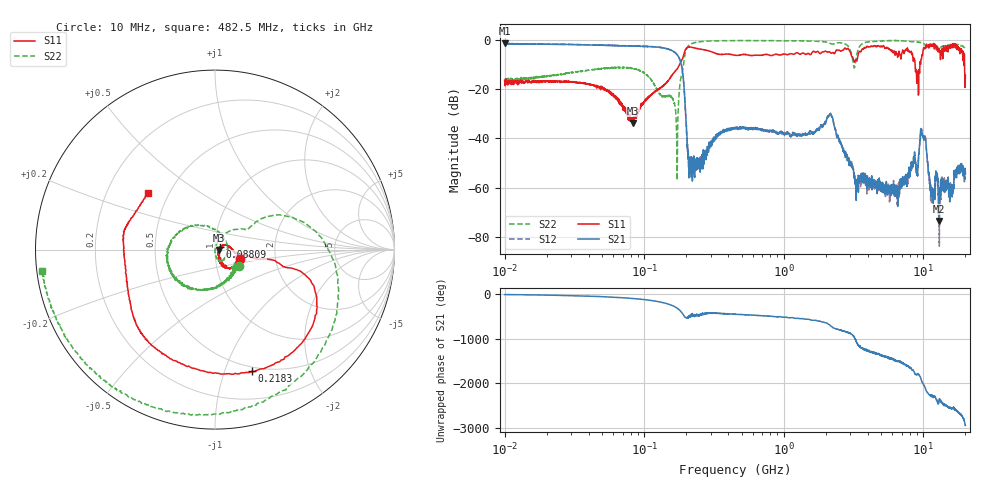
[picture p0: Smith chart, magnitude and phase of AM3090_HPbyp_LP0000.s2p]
# Hz S DB R 50
!freq MagS11 AngS11 MagS21 AngS21 MagS12 AngS12 MagS22 AngS22
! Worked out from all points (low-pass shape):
!   3201 points, 10 MHz to 20 GHz, reference 50 ohm
!   highest |S21| = -1.39 dB at 10.05 MHz (marker M1); lowest = -73.5 dB at 12.95 GHz (marker M2)
!   |S21| within 3 dB of the highest: start of sweep to 158.6 MHz
!   lowest |S11| = -33.7 dB at 82.62 MHz (marker M3), VSWR 1.04, Z = 52.1 - j0.2 ohm
!   |S11| at or under -10 dB: start of sweep to 179.1 MHz; 8.727 GHz to 9.453 GHz (725.5 MHz wide, 7.98 % of centre); 19.73 GHz to end of sweep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
!   |S22| runs from -57.0 to -0.2 dB; largest |S21 - S12| = 0.04
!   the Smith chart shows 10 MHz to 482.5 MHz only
!   S11 on the Smith chart (normalised r, x): 10 MHz: 1.32, -0.13; 88.09 MHz: 1.05, +0.03; 218.3 MHz: 0.46, -1.25; 482.5 MHz: 0.38, +0.32
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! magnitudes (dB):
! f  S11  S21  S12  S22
! 10 MHz  -16.5  -1.5  -1.7  -15.8
! 10.05 MHz  -16.9  -1.4  -1.5  -17.2
! 35.55 MHz  -17.6  -2.0  -1.9  -12.7
! 82.62 MHz  -33.7  -2.5  -2.5  -11.6
! 88.09 MHz  -30.5  -2.5  -2.5  -12.0
! 126.1 MHz  -20.2  -2.9  -3.0  -21.2
! 169.7 MHz  -12.2  -5.6  -5.5  -33.3
! 181.8 MHz  -9.2  -8.6  -8.6  -16.4
! 207.2 MHz  -2.9  -48.0  -48.6  -2.5
! 218.3 MHz  -3.0  -52.0  -51.1  -1.6
! 447.2 MHz  -6.3  -35.7  -35.8  -0.3
! 482.5 MHz  -6.2  -35.4  -36.0  -0.3
! 1.59 GHz  -5.3  -37.7  -37.7  -0.4
! 2.17 GHz  -5.3  -30.3  -30.0  -1.5
! 3.297 GHz  -8.3  -60.2  -59.0  -7.5
! 5.639 GHz  -3.7  -61.2  -60.2  -0.3
! 9.09 GHz  -14.4  -55.3  -51.8  -0.9
! 9.901 GHz  -5.2  -38.9  -39.1  -1.3
! 11.47 GHz  -2.7  -62.5  -62.4  -1.9
! 12.95 GHz  -3.4  -73.5  -67.8  -3.4
! 17.14 GHz  -2.3  -54.6  -54.6  -1.8
! 20 GHz  -14.4  -54.4  -53.7  -3.7
